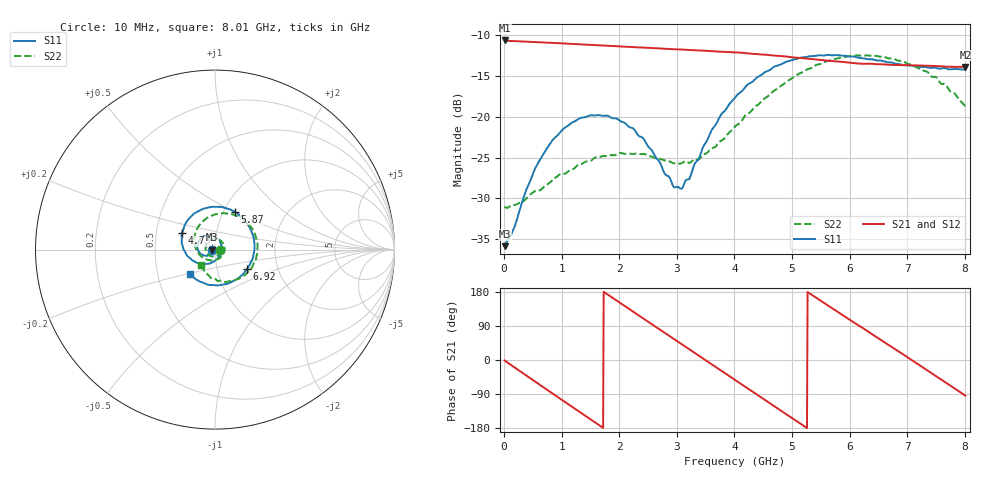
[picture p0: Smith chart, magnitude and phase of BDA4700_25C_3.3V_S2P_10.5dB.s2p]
!Agilent Technologies,E5071B,MY42404982,A.09.10
!Date: Mon Oct 20 18:07:25 2025
!Data & Calibration Information:
!Freq	S11:SOLT2(ON)	S21:SOLT2(ON)	S12:SOLT2(ON)	S22:SOLT2(ON)
# Hz S RI R 50
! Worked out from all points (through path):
!   801 points, 10 MHz to 8.01 GHz, reference 50 ohm
!   highest |S21| = -10.61 dB at 20 MHz (marker M1); lowest = -13.9 dB at 8.01 GHz (marker M2)
!   group delay of S21, straight-line fit = 282 ps
!   lowest |S11| = -35.9 dB at 10 MHz (marker M3), VSWR 1.03, Z = 48.4 - j0.115 ohm
!   |S11| at or under -10 dB: start of sweep to end of sweep
!   |S22| runs from -31.2 to -12.4 dB; largest |S21 - S12| = 0.0035
!   S11 on the Smith chart (normalised r, x): 10 MHz: 0.97, -0.00; 4.73 GHz: 0.68, +0.13; 5.87 GHz: 1.13, +0.50; 6.92 GHz: 1.40, -0.31; 8.01 GHz: 0.73, -0.21
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1e7  -0.0161 -0.00118  0.2946 -0.00624  0.2947 -0.00682  0.0282 -0.00145
2e7  -0.0165 -0.00197  0.2945 -0.0115  0.2944 -0.0125  0.0279 -0.00165
3.4e8  -0.0236 -0.0217  0.2347 -0.1709  0.2345 -0.171  0.0222 -0.0211
7.2e8  -0.0519 -0.0343  0.0705 -0.2773  0.0708 -0.2772  -0.00212 -0.0378
1.02e9  -0.0806 -0.0232  -0.0818 -0.2707  -0.0817 -0.2708  -0.0293 -0.0337
1.35e9  -0.0987 0.0092  -0.2166 -0.1759  -0.2167 -0.176  -0.0512 -0.00534
1.93e9  -0.0654 0.0732  -0.2546 0.0958  -0.2546 0.0959  -0.0251 0.0527
2.32e9  -0.0138 0.0765  -0.1319 0.2327  -0.1318 0.2326  0.0209 0.0557
2.68e9  0.0272 0.0468  0.0328 0.2615  0.0323 0.2615  0.0508 0.0221
2.94e9  0.0364 0.00907  0.1439 0.2173  0.1438 0.2167  0.0511 -0.0101
3.08e9  0.0339 -0.0131  0.1925 0.1735  0.1907 0.1748  0.0439 -0.0278
3.53e9  -0.0153 -0.0707  0.2538 -0.0153  0.254 -0.0157  -0.00803 -0.06
4.01e9  -0.1124 -0.0677  0.1519 -0.1973  0.1521 -0.1968  -0.0796 -0.0354
4.37e9  -0.1721 -0.00439  0.00398 -0.2435  0.00396 -0.2439  -0.1138 0.0248
4.73e9  -0.1846 0.0909  -0.1394 -0.1924  -0.1385 -0.1929  -0.105 0.104
5.35e9  -0.0614 0.2281  -0.2238 0.0346  -0.224 0.0332  0.024 0.1992
5.87e9  0.1095 0.2114  -0.1065 0.1901  -0.1062 0.1894  0.1734 0.1539
6.28e9  0.2007 0.1073  0.0391 0.2083  0.0418 0.207  0.2353 0.0388
6.68e9  0.2143 -0.0309  0.1619 0.1326  0.1622 0.1323  0.2136 -0.0821
6.92e9  0.1801 -0.1054  0.2001 0.0561  0.2 0.0552  0.1705 -0.14
7.47e9  0.0221 -0.1996  0.1584 -0.1307  0.1583 -0.131  0.0196 -0.1755
8.01e9  -0.1394 -0.138  -0.0149 -0.2018  -0.0144 -0.2021  -0.078 -0.0862
